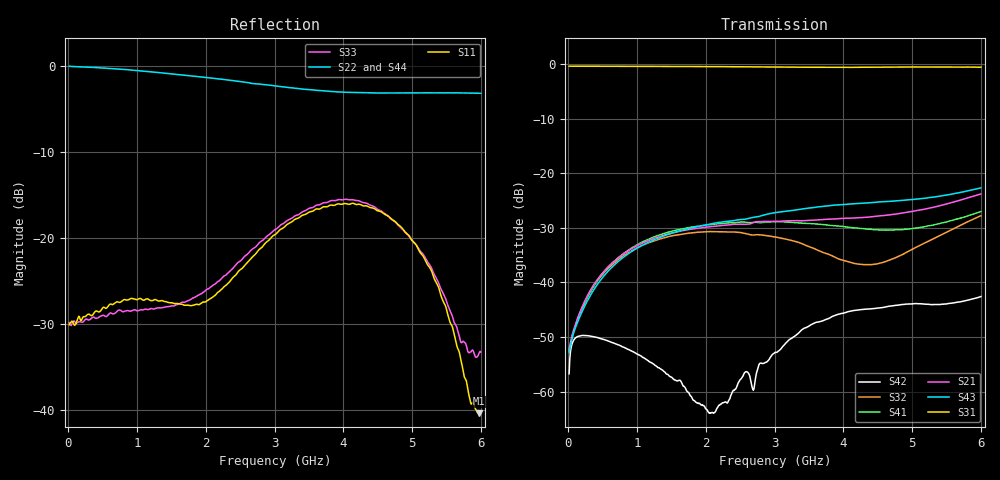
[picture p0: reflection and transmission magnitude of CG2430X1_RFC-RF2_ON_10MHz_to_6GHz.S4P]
!CEL
!CG2430X1
!Port1: RFC Port2: RF1  Port3: RF2 Port4: RF3
!Data & Calibration Information:
!Freq	S11:SOLT4(ON)	S12:SOLT4(ON)	S13:SOLT4(ON)	S14:SOLT4(ON)
!	S21:SOLT4(ON)	S22:SOLT4(ON)	S23:SOLT4(ON)	S24:SOLT4(ON)
!	S31:SOLT4(ON)	S32:SOLT4(ON)	S33:SOLT4(ON)	S34:SOLT4(ON)
!	S41:SOLT4(ON)	S42:SOLT4(ON)	S43:SOLT4(ON)	S44:SOLT4(ON)
# Hz S dB R 50
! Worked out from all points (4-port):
!   600 points, 10 MHz to 6 GHz, reference 50 ohm
!   strongest paths, dB at 10 MHz, 1.51 GHz, 3.01 GHz, 4.51 GHz, 6 GHz:
!     S31: -0.4, -0.4, -0.5, -0.5, -0.5
!     S43: -52.8, -30.9, -27.2, -25.3, -22.7
!     S21: -52.3, -30.9, -28.8, -27.8, -23.8
!     S41: -52.5, -30.6, -28.9, -30.4, -27.0
!     S32: -52.8, -31.4, -31.7, -36.5, -27.8
!     S42: -56.8, -57.5, -52.8, -44.7, -42.6
!   lowest |S11| = -40.4 dB at 5.97 GHz (marker M1), VSWR 1.02, Z = 50.7 - j0.675 ohm
!   |S11| at or under -10 dB: start of sweep to end of sweep
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1e7  -30.12 0.7  -52.32 12.5  -0.36 -0.2  -52.53 12.0
     -52.32 13.3  -0.07 -0.6  -52.70 13.7  -56.80 50.8
     -0.36 -0.2  -52.75 13.0  -29.87 -1.6  -52.89 12.0
     -52.54 12.6  -56.75 50.8  -52.84 13.0  -0.09 -0.5
1.36e9  -27.30 19.3  -31.43 57.2  -0.40 -12.0  -31.13 39.8
        -31.43 57.3  -0.85 -56.6  -31.93 39.8  -56.00 -40.1
        -0.41 -12.0  -31.93 39.7  -28.13 26.6  -31.62 61.7
        -31.15 39.8  -55.99 -40.2  -31.61 61.7  -0.79 -56.8
2.1e9  -26.90 39.3  -29.75 52.2  -0.44 -18.2  -29.38 19.3
       -29.74 52.2  -1.47 -84.0  -30.67 19.9  -63.82 -115.0
       -0.44 -18.2  -30.67 19.9  -25.55 31.4  -29.22 56.6
       -29.36 19.0  -63.86 -112.3  -29.19 56.6  -1.42 -83.8
4.24e9  -16.13 44.3  -28.16 61.3  -0.56 -35.6  -30.09 -57.7
        -28.12 60.9  -3.15 -165.1  -36.71 -87.2  -44.96 110.7
        -0.56 -35.6  -36.67 -88.1  -15.76 45.7  -25.56 47.9
        -30.10 -57.3  -45.00 110.2  -25.51 47.6  -3.03 -163.3
5.26e9  -23.52 36.9  -26.27 74.2  -0.49 -44.8  -29.64 -99.6
        -26.36 73.6  -3.17 166.4  -32.30 -162.8  -44.09 84.8
        -0.50 -44.8  -32.30 -163.7  -23.22 26.3  -24.44 48.0
        -29.58 -100.5  -44.05 84.4  -24.43 48.0  -3.04 171.3
5.97e9  -40.41 -44.2  -23.97 78.4  -0.56 -52.0  -27.16 -127.2
        -23.90 77.9  -3.21 152.6  -28.37 176.4  -42.76 76.6
        -0.56 -52.0  -27.93 175.7  -33.49 -45.9  -22.72 48.0
        -27.12 -125.9  -42.72 76.1  -22.74 48.4  -3.23 158.3
6e9  -40.23 -53.4  -23.86 78.1  -0.56 -52.4  -27.02 -128.3
     -23.78 78.0  -3.22 152.0  -28.21 175.6  -42.65 76.0
     -0.53 -52.4  -27.78 175.1  -33.28 -47.0  -22.63 47.7
     -27.00 -126.8  -42.59 75.5  -22.67 48.3  -3.25 157.5
